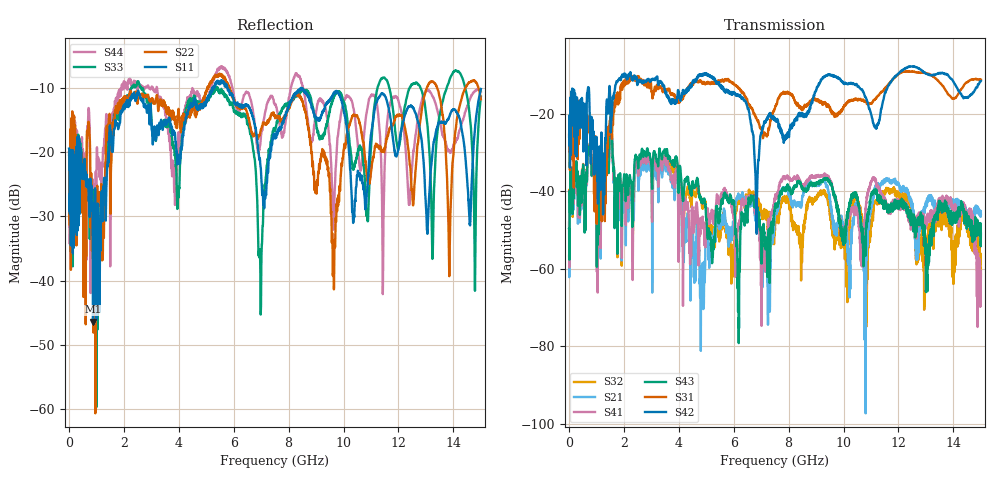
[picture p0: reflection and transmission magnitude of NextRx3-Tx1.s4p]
! FILE: N:\QM 2007\Prüfprotokolle\Highspeed\Konfektionierte Ltg\L45593-D106\D30\8216\0002\Next  Platine 1\NextRx3-Tx1.s4p
# MHz S DB R 50.00
! FREQ  S11  S12  S13  S14
!  S21  S22  S23  S24
!  S31  S32  S33  S34
!  S41  S42  S43  S44
!  DB  ANG  DB  ANG  DB  ANG  DB  ANG
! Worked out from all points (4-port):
!   2999 points, 10 MHz to 15 GHz, reference 50 ohm
!   strongest paths, dB at 10 MHz, 3.755 GHz, 7.505 GHz, 11.26 GHz, 15 GHz:
!     S42: -25.9, -16.3, -21.4, -22.7, -11.6
!     S31: -25.3, -15.1, -18.6, -15.4, -11.2
!     S43: -49.6, -33.0, -44.0, -41.4, -50.9
!     S41: -56.6, -37.5, -41.5, -39.0, -61.9
!     S21: -48.2, -37.9, -45.5, -38.5, -45.9
!     S32: -48.0, -34.3, -50.1, -42.4, -61.2
!   lowest |S11| = -46.4 dB at 880 MHz (marker M1), VSWR 1.01, Z = 49.6 - j0.288 ohm
!   |S11| at or under -10 dB: start of sweep to 5.215 GHz; 5.775 GHz to 8.449 GHz (2.674 GHz wide, 37.6 % of centre); 8.453 GHz to end of sweep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
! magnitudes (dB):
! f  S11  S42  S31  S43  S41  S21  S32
! 10 MHz  -19.4  -25.9  -25.3  -49.6  -56.6  -48.2  -48.0
! 880 MHz  -46.4  -28.2  -29.0  -34.5  -33.8  -34.1  -34.5
! 3.53 GHz  -15.6  -14.7  -14.1  -30.9  -33.2  -34.9  -32.5
! 4.845 GHz  -12.5  -9.9  -12.0  -42.7  -46.9  -62.5  -43.7
! 6.835 GHz  -17.3  -51.0  -21.3  -44.1  -44.8  -45.7  -42.9
! 9.635 GHz  -10.8  -10.5  -20.1  -40.5  -40.1  -48.2  -51.4
! 15 GHz  -10.2  -11.6  -11.2  -50.9  -61.9  -45.9  -61.2
